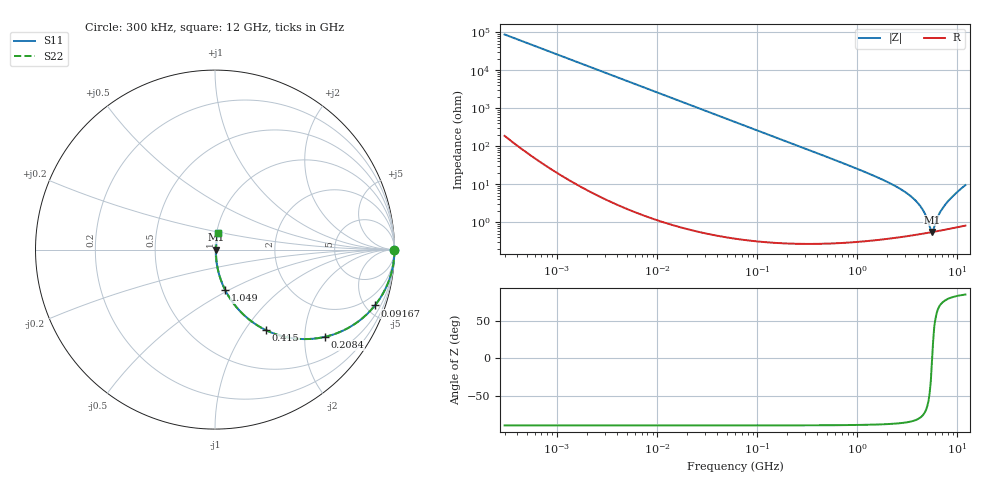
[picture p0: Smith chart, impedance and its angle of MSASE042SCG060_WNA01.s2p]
! MSASE042SCG060_WNA01  S-PARAMETER MODEL  ( General Type )
! Model Generated by TAIYO YUDEN Corporation (http://www.ty-top.com)
! Version 1.0
! TAIYO YUDEN Control No. 130801
! Copyright(c) 2013 TAIYO YUDEN CO.,LTD. All Rights Reserved.
! Product Description (link to TY-COMPAS)
! https://ds.yuden.co.jp/TYCOMPAS/or/detail?pn=MSASE042SCG060BWNA01&u=M
! Products Name : Multilayer Ceramic Capacitors
! Characteristics :
!  Capacitance : 6 pF , Rated Voltage : 16V , TCC : CG / C0G
!  Case Size : 0.4 x 0.2 / 0.016 x 0.008 [mm/inch] , Thickness : 0.2 / 0.008 [mm/inch]
!  (Conditions: Temperature = 25 degC , DC Bias Current/Voltage = 0A / 0V)
! External Node Assignments :
!  1  o---| |---o  2
! GND o---------o GND
! Frequency Range : 0.3MHz  -  12000MHz  [ 401 STEP ]
# MHz S RI R 50
! Freq[MHz].  S11 Real  S11 Imag  S21 Real  S21 Imag  S12 Real  S12 Imag  S22 Real  S22 Imag
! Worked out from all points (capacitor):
!   401 points, 300 kHz to 12 GHz, reference 50 ohm
!   read as one part in series: C = 6.06 pF near 316.3 kHz
!   lowest |Z| = 552 mohm at 5.566 GHz (marker M1)
!   series resonance near 5.589 GHz, so ESL is about 130 pH
!   S11 on the Smith chart (normalised r, x): 300 kHz: open; 91.67 MHz: 1.01, -5.73; 208.4 MHz: 1.01, -2.52; 415 MHz: 1.01, -1.26; 1.049 GHz: 1.01, -0.48; 12 GHz: 1.02, +0.19
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0.3  1 -0.00114  3.75e-06 0.00114  3.75e-06 0.00114  1 -0.00114
1.769972  1 -0.00674  4.92e-05 0.00674  4.92e-05 0.00674  1 -0.00674
10.44266  0.9984 -0.0397  0.0016 0.0397  0.0016 0.0397  0.9984 -0.0397
27.82928  0.9888 -0.1048  0.0112 0.1048  0.0112 0.1048  0.9888 -0.1048
60  0.9502 -0.2171  0.0498 0.2171  0.0498 0.2171  0.9502 -0.2171
91.67136  0.8911 -0.311  0.1089 0.311  0.1089 0.311  0.8911 -0.311
208.3979  0.6128 -0.486  0.3872 0.486  0.3872 0.486  0.6128 -0.486
353.9943  0.3537 -0.4763  0.6463 0.4763  0.6463 0.4763  0.3537 -0.4763
414.98  0.2846 -0.4491  0.7154 0.4491  0.7154 0.4491  0.2846 -0.4491
651.0506  0.1385 -0.3419  0.8615 0.3419  0.8615 0.3419  0.1385 -0.3419
1048.836  0.0577 -0.227  0.9423 0.227  0.9423 0.227  0.0577 -0.227
2088.533  0.0152 -0.1063  0.9848 0.1063  0.9848 0.1063  0.0152 -0.1063
3026.31  0.00794 -0.0607  0.9921 0.0607  0.9921 0.0607  0.00794 -0.0607
3944.255  0.00581 -0.0333  0.9942 0.0333  0.9942 0.0333  0.00581 -0.0333
4623.766  0.00535 -0.018  0.9946 0.018  0.9946 0.018  0.00535 -0.018
5278.635  0.00537 -0.00558  0.9946 0.00558  0.9946 0.00558  0.00537 -0.00558
5565.855  0.00547 -0.000418  0.9945 0.000418  0.9945 0.000418  0.00547 -0.000418
5868.704  0.00564 0.00512  0.9944 -0.00512  0.9944 -0.00512  0.00564 0.00512
6699.894  0.00628 0.0173  0.9937 -0.0173  0.9937 -0.0173  0.00628 0.0173
7648.807  0.00725 0.0293  0.9927 -0.0293  0.9927 -0.0293  0.00725 0.0293
9968.853  0.0111 0.0613  0.9889 -0.0613  0.9889 -0.0613  0.0111 0.0613
12000  0.0168 0.0924  0.9832 -0.0924  0.9832 -0.0924  0.0168 0.0924
